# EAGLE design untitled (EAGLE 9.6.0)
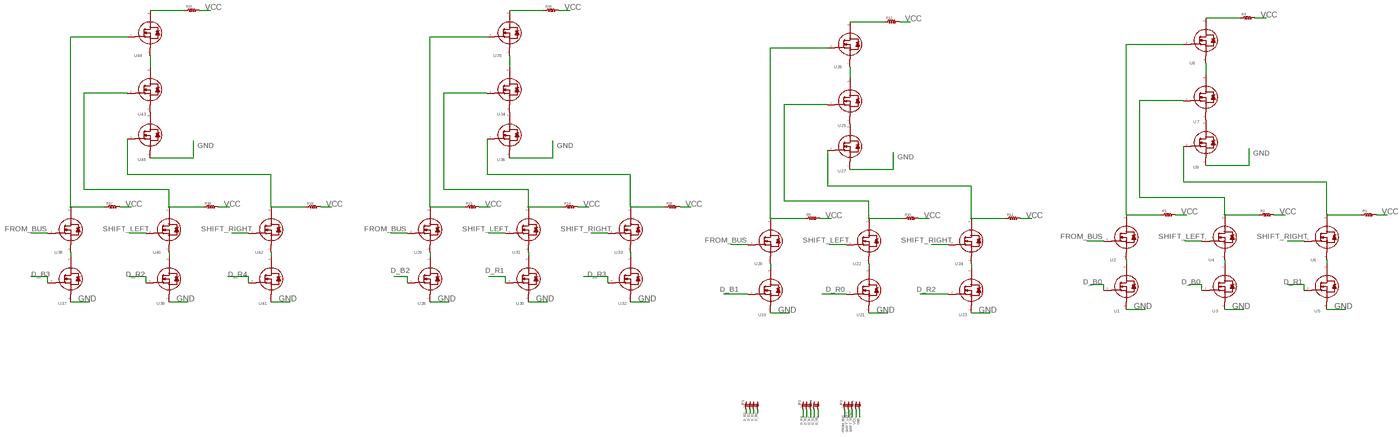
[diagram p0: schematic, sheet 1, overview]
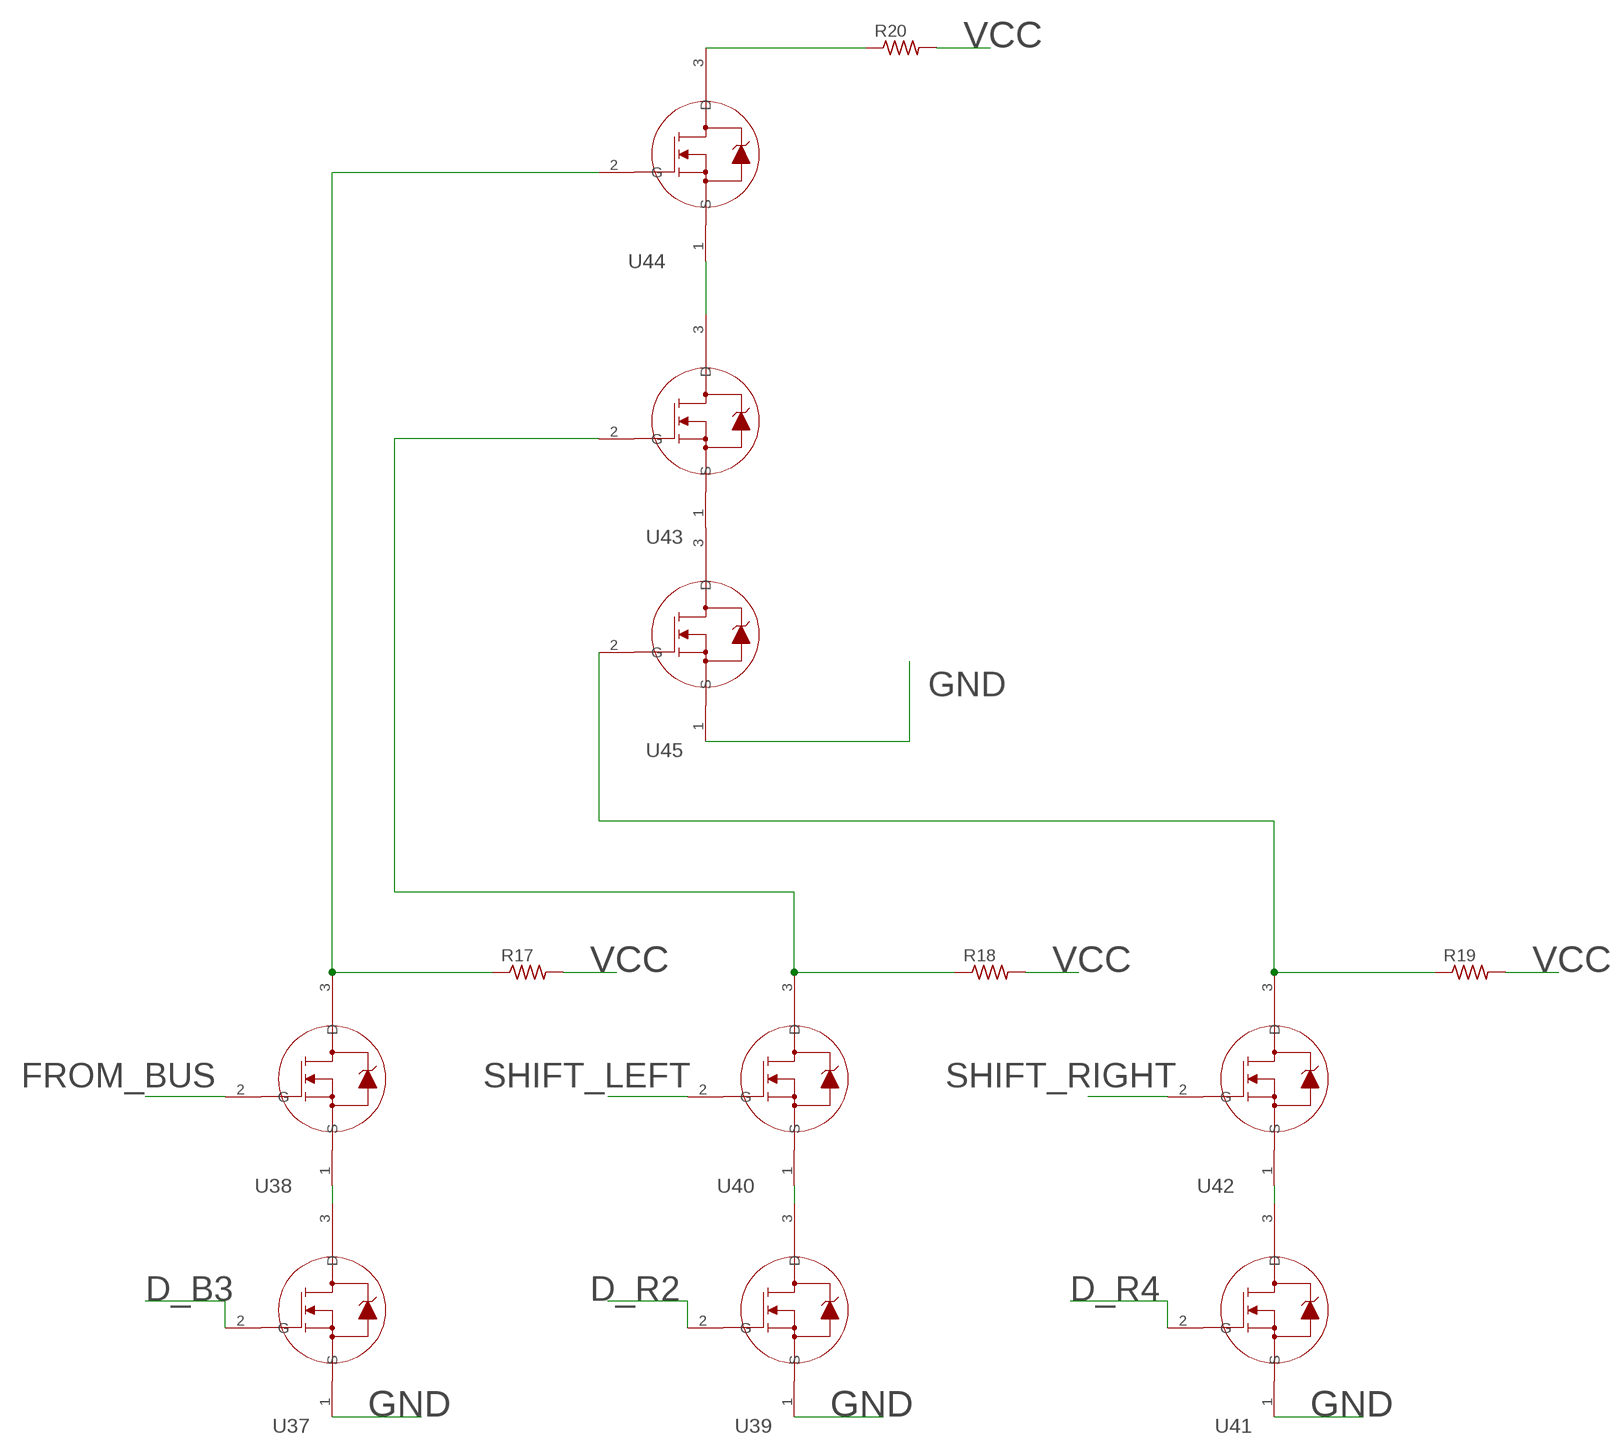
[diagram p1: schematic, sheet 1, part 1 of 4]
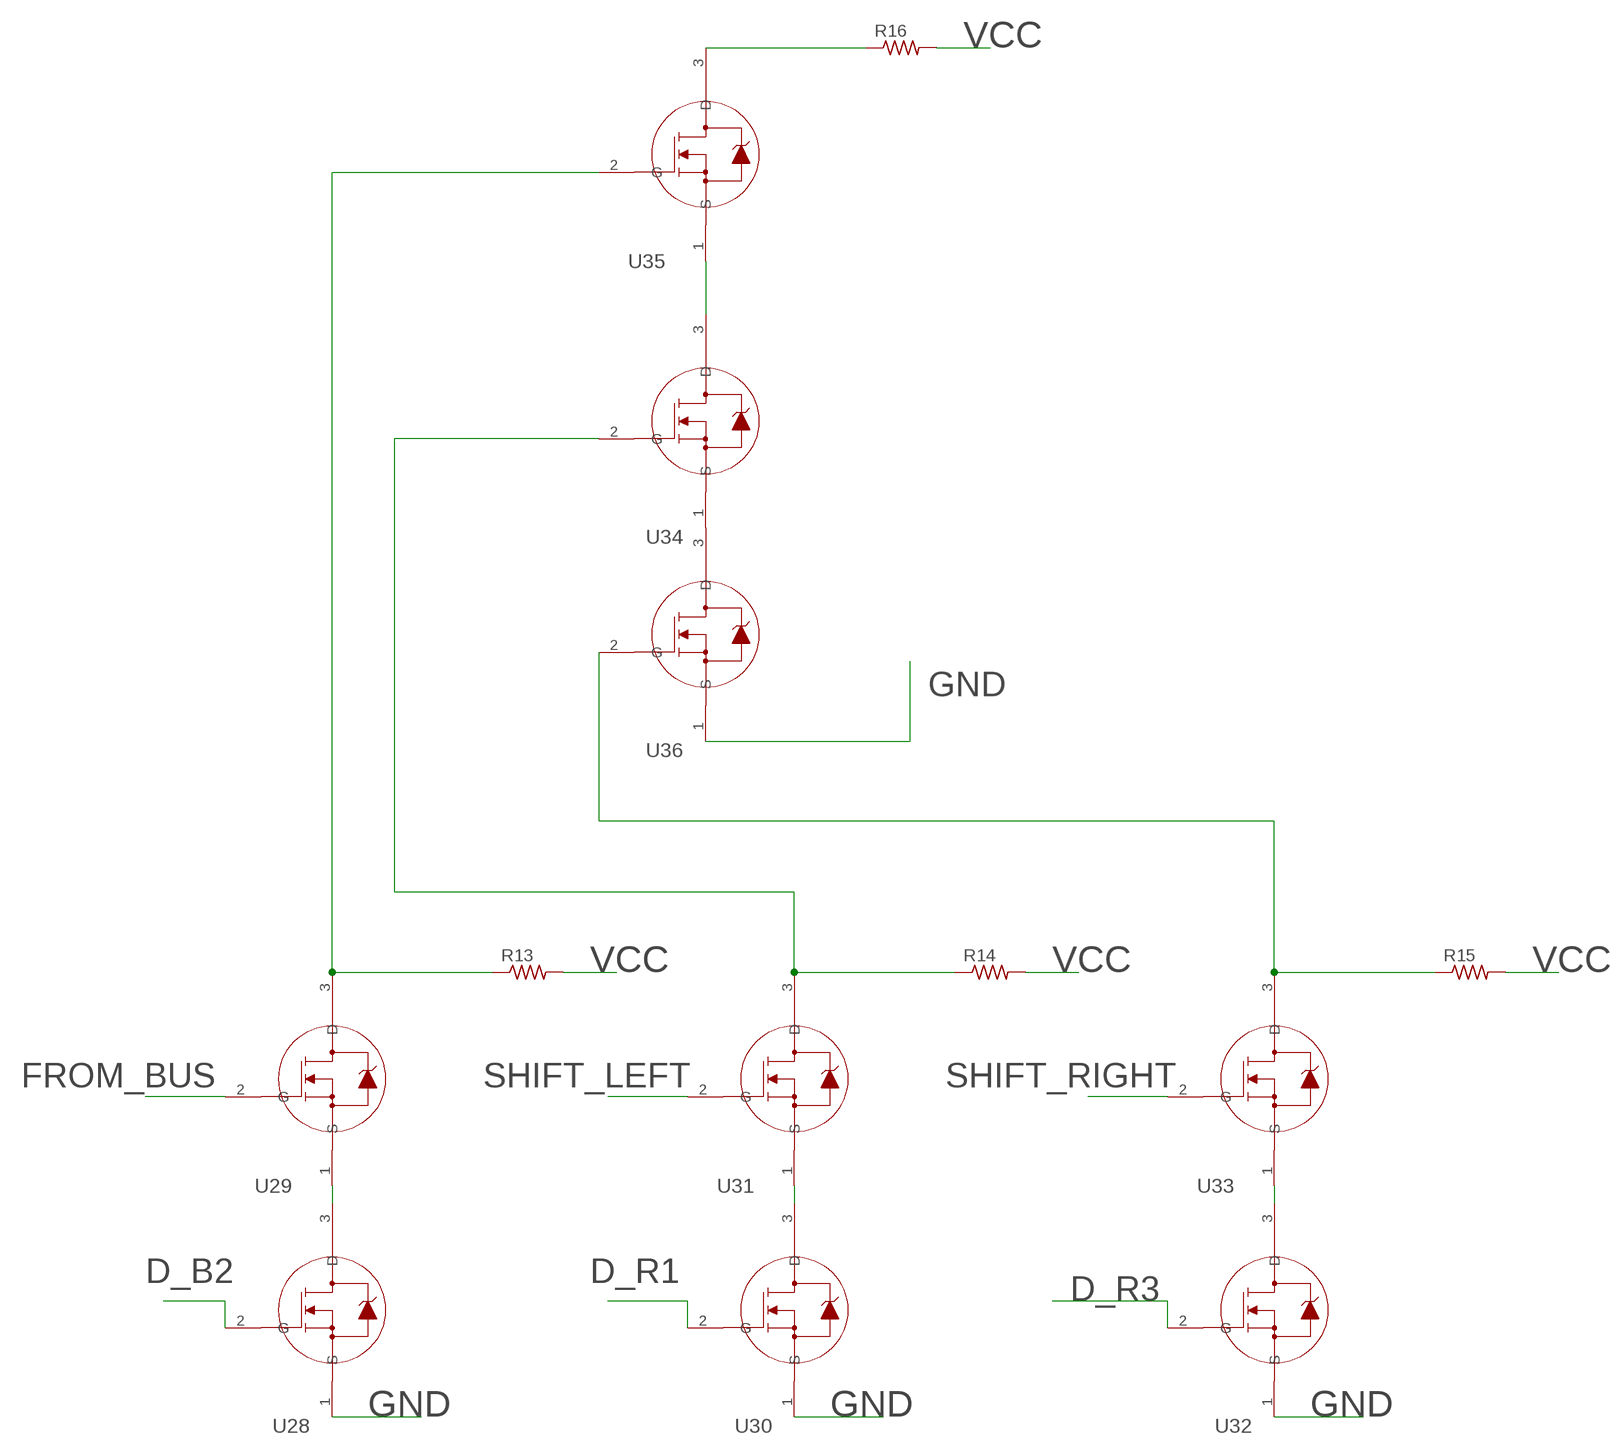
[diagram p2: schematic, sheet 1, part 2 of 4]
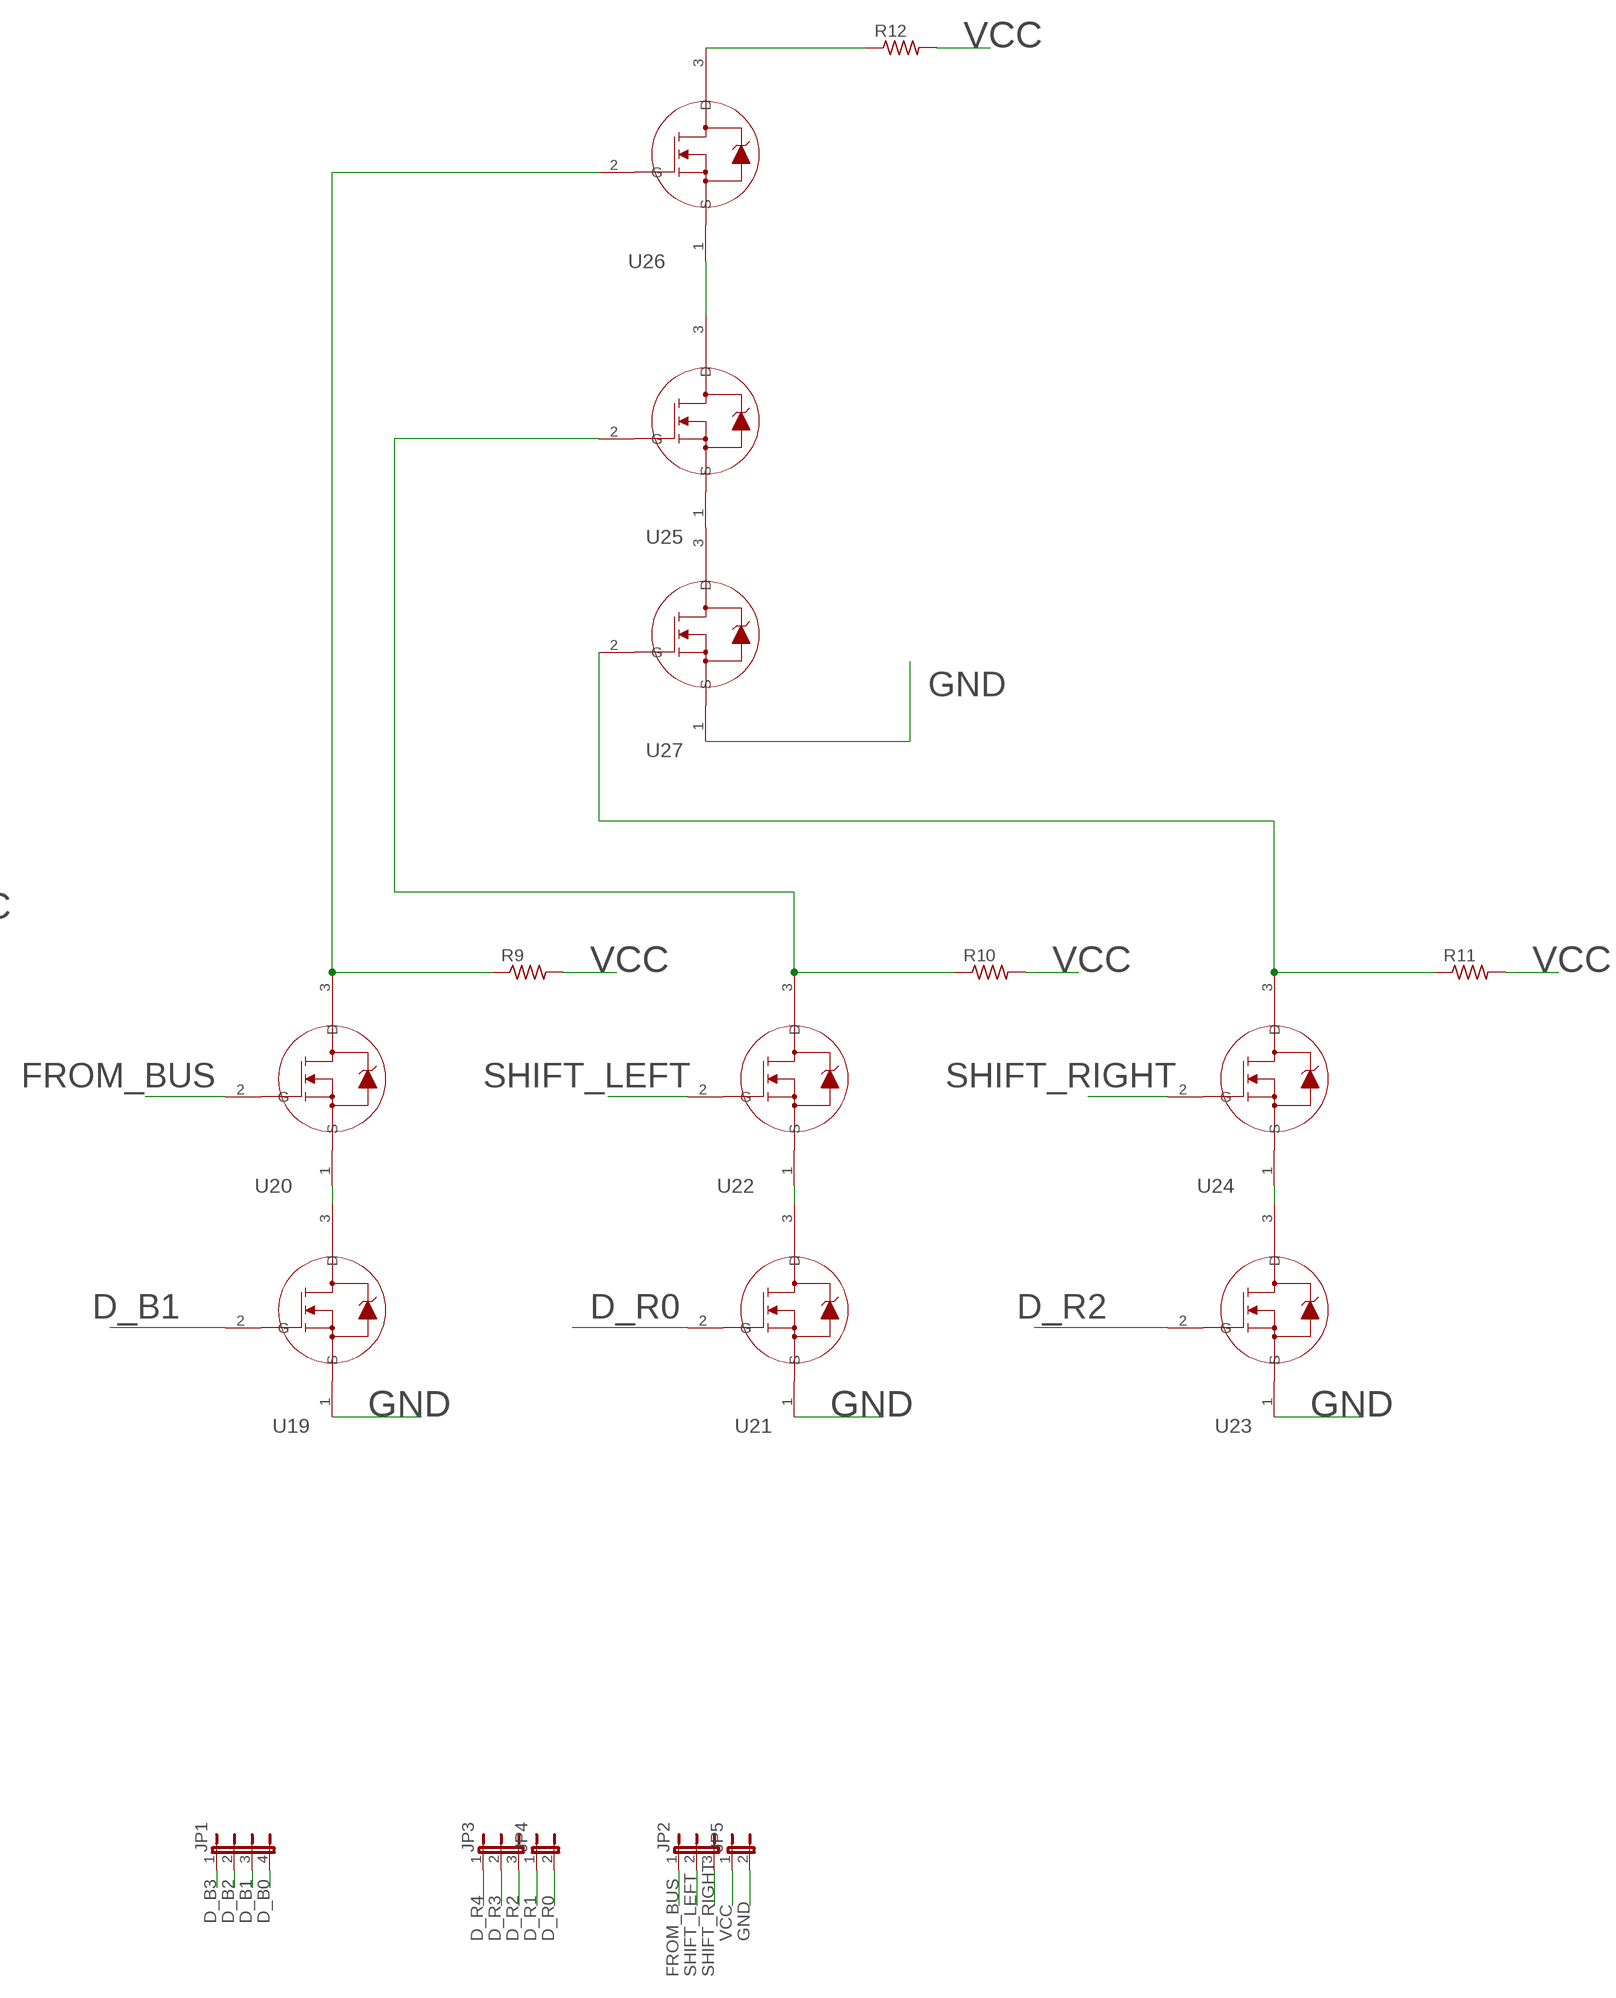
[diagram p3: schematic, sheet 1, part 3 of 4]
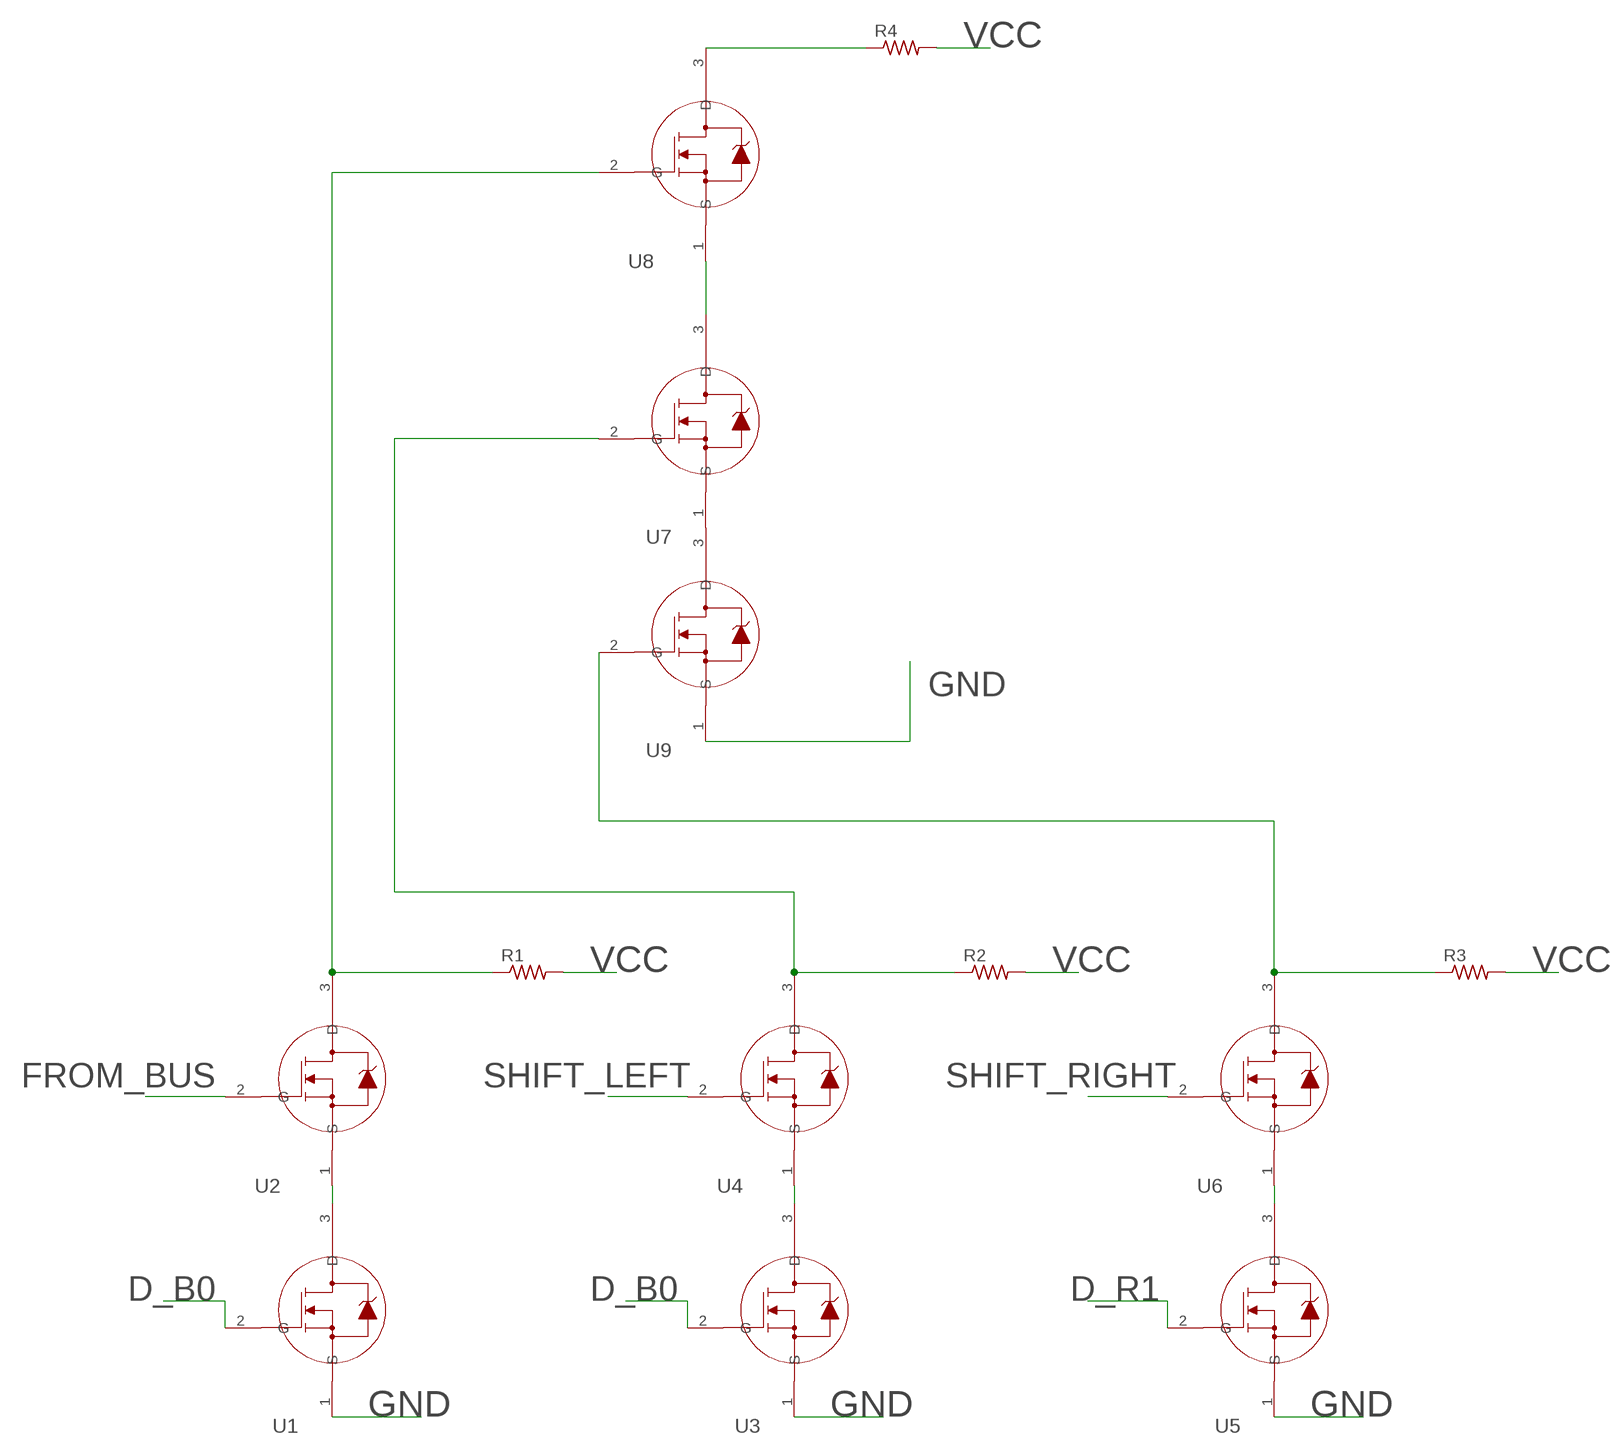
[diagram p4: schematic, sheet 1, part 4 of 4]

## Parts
JP1  JP4E  [JP4]
JP2  JP2E  [JP2]
JP3  JP2E  [JP2]
JP4  JP1E  [JP1]
JP5  JP1E  [JP1]
R1  R-US_0204/7  [0204/7]
R2  R-US_0204/7  [0204/7]
R3  R-US_0204/7  [0204/7]
R4  R-US_0204/7  [0204/7]
R9  R-US_0204/7  [0204/7]
R10  R-US_0204/7  [0204/7]
R11  R-US_0204/7  [0204/7]
R12  R-US_0204/7  [0204/7]
R13  R-US_0204/7  [0204/7]
R14  R-US_0204/7  [0204/7]
R15  R-US_0204/7  [0204/7]
R16  R-US_0204/7  [0204/7]
R17  R-US_0204/7  [0204/7]
R18  R-US_0204/7  [0204/7]
R19  R-US_0204/7  [0204/7]
R20  R-US_0204/7  [0204/7]
U1  2N7000RLRAG  [TO-92_ONS]
U2  2N7000RLRAG  [TO-92_ONS]
U3  2N7000RLRAG  [TO-92_ONS]
U4  2N7000RLRAG  [TO-92_ONS]
U5  2N7000RLRAG  [TO-92_ONS]
U6  2N7000RLRAG  [TO-92_ONS]
U7  2N7000RLRAG  [TO-92_ONS]
U8  2N7000RLRAG  [TO-92_ONS]
U9  2N7000RLRAG  [TO-92_ONS]
U19  2N7000RLRAG  [TO-92_ONS]
U20  2N7000RLRAG  [TO-92_ONS]
U21  2N7000RLRAG  [TO-92_ONS]
U22  2N7000RLRAG  [TO-92_ONS]
U23  2N7000RLRAG  [TO-92_ONS]
U24  2N7000RLRAG  [TO-92_ONS]
U25  2N7000RLRAG  [TO-92_ONS]
U26  2N7000RLRAG  [TO-92_ONS]
U27  2N7000RLRAG  [TO-92_ONS]
U28  2N7000RLRAG  [TO-92_ONS]
U29  2N7000RLRAG  [TO-92_ONS]
U30  2N7000RLRAG  [TO-92_ONS]
U31  2N7000RLRAG  [TO-92_ONS]
U32  2N7000RLRAG  [TO-92_ONS]
U33  2N7000RLRAG  [TO-92_ONS]
U34  2N7000RLRAG  [TO-92_ONS]
U35  2N7000RLRAG  [TO-92_ONS]
U36  2N7000RLRAG  [TO-92_ONS]
U37  2N7000RLRAG  [TO-92_ONS]
U38  2N7000RLRAG  [TO-92_ONS]
U39  2N7000RLRAG  [TO-92_ONS]
U40  2N7000RLRAG  [TO-92_ONS]
U41  2N7000RLRAG  [TO-92_ONS]
U42  2N7000RLRAG  [TO-92_ONS]
U43  2N7000RLRAG  [TO-92_ONS]
U44  2N7000RLRAG  [TO-92_ONS]
U45  2N7000RLRAG  [TO-92_ONS]

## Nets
D_B0: JP1.4 U1.2(G) U3.2(G)
D_B1: JP1.3 U19.2(G)
D_B2: JP1.2 U28.2(G)
D_B3: JP1.1 U37.2(G)
D_R0: JP4.2 U21.2(G)
D_R1: JP4.1 U5.2(G) U30.2(G)
D_R2: JP3.3 U23.2(G) U39.2(G)
D_R3: JP3.2 U32.2(G)
D_R4: JP3.1 U41.2(G)
FROM_BUS: JP2.1 U2.2(G) U20.2(G) U29.2(G) U38.2(G)
GND: JP5.2 U1.1(S) U3.1(S) U5.1(S) U9.1(S) U19.1(S) U21.1(S) U23.1(S) U27.1(S) U28.1(S) U30.1(S) U32.1(S) U36.1(S) U37.1(S) U39.1(S) U41.1(S) U45.1(S)
N$1: U1.3(D) U2.1(S)
N$2: R1.1 U2.3(D) U8.2(G)
N$3: U3.3(D) U4.1(S)
N$4: R2.1 U4.3(D) U7.2(G)
N$5: U5.3(D) U6.1(S)
N$6: R3.1 U6.3(D) U9.2(G)
N$7: U7.3(D) U8.1(S)
N$9: R4.1 U8.3(D)
N$11: U7.1(S) U9.3(D)
N$19: U19.3(D) U20.1(S)
N$20: R9.1 U20.3(D) U26.2(G)
N$21: U21.3(D) U22.1(S)
N$22: R10.1 U22.3(D) U25.2(G)
N$23: U23.3(D) U24.1(S)
N$24: R11.1 U24.3(D) U27.2(G)
N$25: U25.3(D) U26.1(S)
N$26: R12.1 U26.3(D)
N$27: U25.1(S) U27.3(D)
N$28: U28.3(D) U29.1(S)
N$29: R13.1 U29.3(D) U35.2(G)
N$30: U30.3(D) U31.1(S)
N$31: R14.1 U31.3(D) U34.2(G)
N$32: U32.3(D) U33.1(S)
N$33: R15.1 U33.3(D) U36.2(G)
N$34: U34.3(D) U35.1(S)
N$35: R16.1 U35.3(D)
N$36: U34.1(S) U36.3(D)
N$37: U37.3(D) U38.1(S)
N$38: R17.1 U38.3(D) U44.2(G)
N$39: U39.3(D) U40.1(S)
N$40: R18.1 U40.3(D) U43.2(G)
N$41: U41.3(D) U42.1(S)
N$42: R19.1 U42.3(D) U45.2(G)
N$43: U43.3(D) U44.1(S)
N$44: R20.1 U44.3(D)
N$45: U43.1(S) U45.3(D)
SHIFT_LEFT: JP2.2 U4.2(G) U22.2(G) U31.2(G) U40.2(G)
SHIFT_RIGHT: JP2.3 U6.2(G) U24.2(G) U33.2(G) U42.2(G)
VCC: JP5.1 R1.2 R2.2 R3.2 R4.2 R9.2 R10.2 R11.2 R12.2 R13.2 R14.2 R15.2 R16.2 R17.2 R18.2 R19.2 R20.2

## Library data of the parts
JP1 = jumper:JP4E: JUMPER
JP2 JP3 = jumper:JP2E: JUMPER
JP4 JP5 = jumper:JP1E: JUMPER
R1-R4 R9-R20 = rcl:R-US_: RESISTOR, American symbol; SPICEPREFIX: R
U1-U9 U19-U45 = Transistor(MOSFET):2N7000RLRAG; COPYRIGHT: Copyright (C) 2022 Ultra Librarian. All rights reserved.; MANUFACTURER_PART_NUMBER: 2N7000RLRAG; MFR_NAME: onsemi

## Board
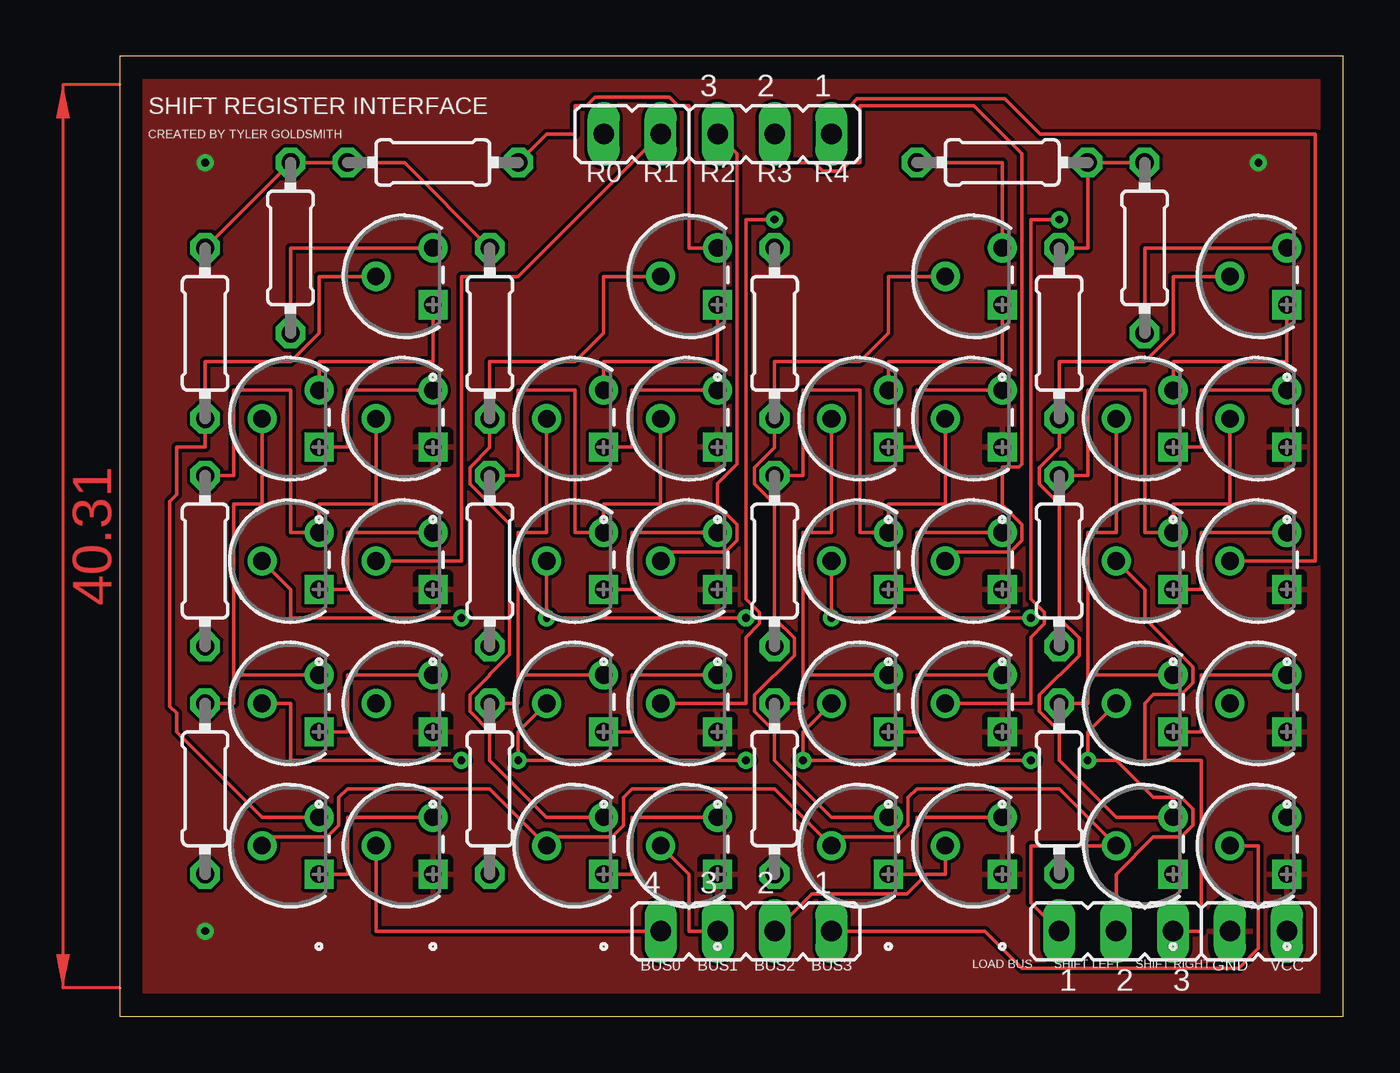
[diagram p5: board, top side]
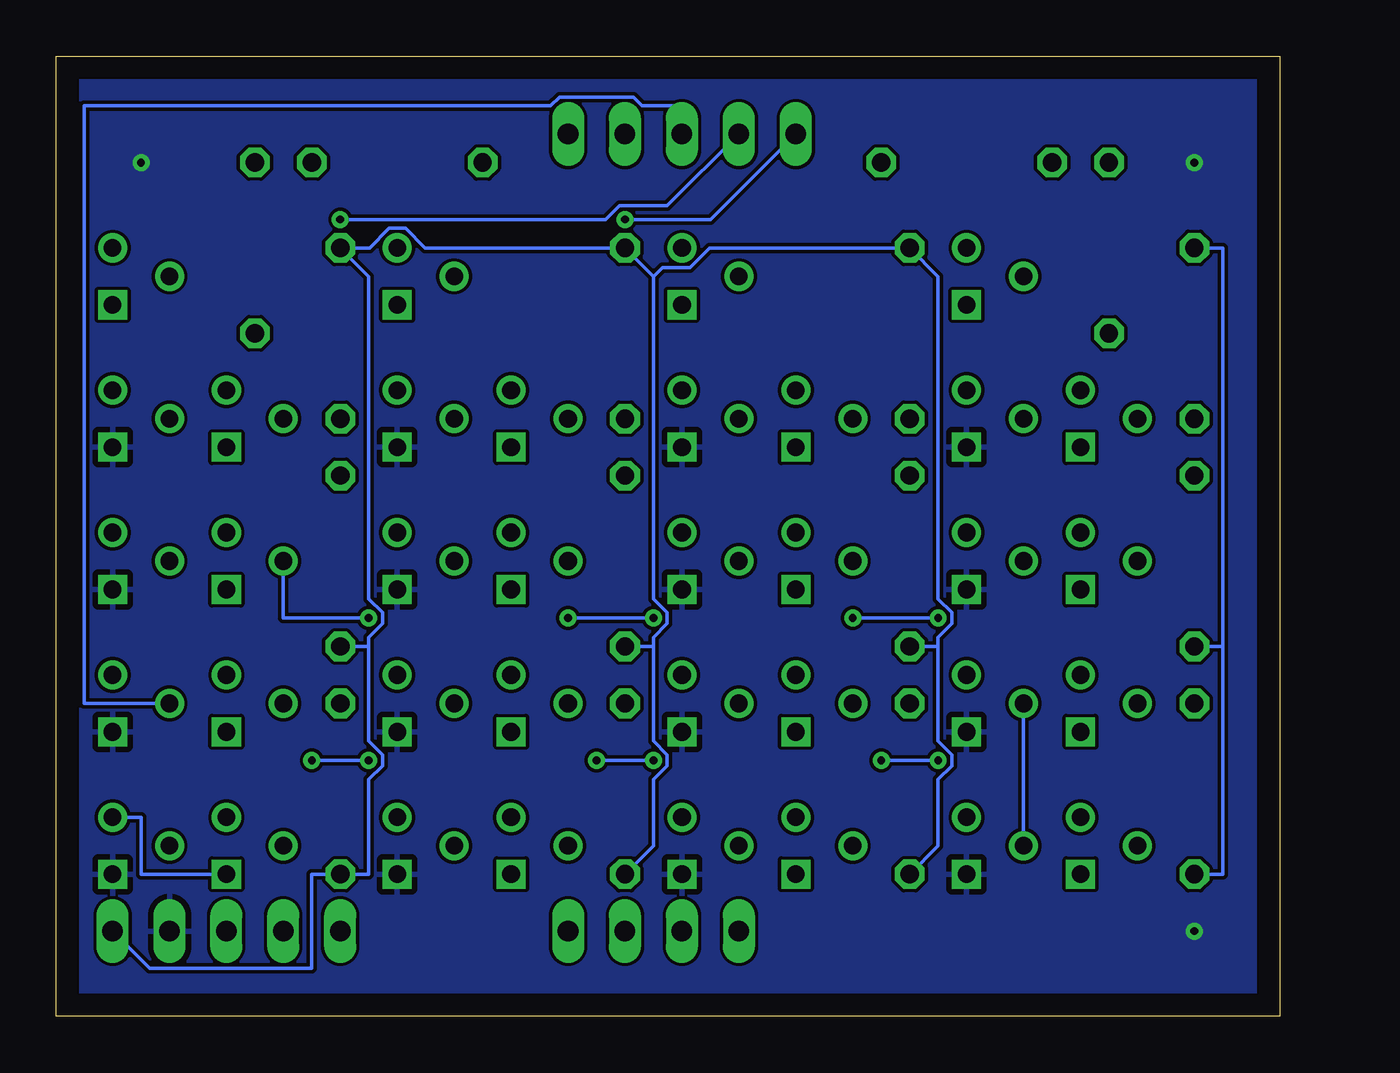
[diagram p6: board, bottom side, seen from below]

Size 54.59 x 42.85 mm. Coordinates in mm from the lower left corner, seen from the top.
Outline: 0,0 54.59,0 54.59,42.85 0,42.85 0,0
Copper layers (1*16): Top 0.035mm / dielectric 1.5mm / Bottom 0.035mm
Design rules "default": minimum track width 6mil, minimum drill 0.35mm, track to track 6mil, track to pad 6mil, pad to pad 6mil, via to via 6mil, smd to smd 6mil, copper to edge 40mil, drill to drill 6mil, minimum pad ring 10mil, minimum via ring 8mil, stop-mask expansion 4mil, vias tented up to drill 0mil, thermal gap 10mil

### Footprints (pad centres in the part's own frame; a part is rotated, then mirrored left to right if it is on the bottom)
JP4 = drill 0.914 long: 1 -3.81,0; 2 -1.27,0; 3 1.27,0; 4 3.81,0
JP2 = drill 0.914 long: 1 -2.54,0; 2 0,0; 3 2.54,0
JP1 = drill 0.914 long: 1 0,-1.27; 2 0,1.27
0204/7 = drill 0.813 octagon: 1 -3.81,0; 2 3.81,0
TO-92_ONS = drill 0.787 pad 1.295 square: 1 0,0 | drill 0.787 pad 1.295: 2 1.27,2.54; 3 2.54,0

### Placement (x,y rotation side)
JP1  27.94,3.81 180 top
JP2  44.45,3.81 0 top
JP3  29.21,39.37 180 top
JP4  22.86,39.37 90 top
JP5  50.8,3.81 90 top
R1  3.81,30.48 90 top
R2  3.81,10.16 270 top
R3  3.81,20.32 270 top
R4  7.62,34.29 90 top
R9  16.51,30.48 90 top
R10  16.51,10.16 270 top
R11  16.51,20.32 270 top
R12  13.97,38.1 180 top
R13  29.21,30.48 90 top
R14  29.21,10.16 270 top
R15  29.21,20.32 270 top
R16  39.37,38.1 0 top
R17  41.91,30.48 90 top
R18  41.91,10.16 270 top
R19  41.91,20.32 270 top
R20  45.72,34.29 90 top
U1  13.97,6.35 90 top
U2  8.89,6.35 90 top
U3  13.97,12.7 90 top
U4  8.89,12.7 90 top
U5  13.97,19.05 90 top
U6  8.89,19.05 90 top
U7  8.89,25.4 90 top
U8  13.97,31.75 90 top
U9  13.97,25.4 90 top
U19  26.67,6.35 90 top
U20  21.59,6.35 90 top
U21  26.67,12.7 90 top
U22  21.59,12.7 90 top
U23  26.67,19.05 90 top
U24  21.59,19.05 90 top
U25  21.59,25.4 90 top
U26  26.67,31.75 90 top
U27  26.67,25.4 90 top
U28  39.37,6.35 90 top
U29  34.29,6.35 90 top
U30  39.37,12.7 90 top
U31  34.29,12.7 90 top
U32  39.37,19.05 90 top
U33  34.29,19.05 90 top
U34  34.29,25.4 90 top
U35  39.37,31.75 90 top
U36  39.37,25.4 90 top
U37  52.07,6.35 90 top
U38  46.99,6.35 90 top
U39  52.07,12.7 90 top
U40  46.99,12.7 90 top
U41  52.07,19.05 90 top
U42  46.99,19.05 90 top
U43  46.99,25.4 90 top
U44  52.07,31.75 90 top
U45  52.07,25.4 90 top

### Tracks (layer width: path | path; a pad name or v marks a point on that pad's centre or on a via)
D_B0
  Top 0.152: U1.2 11.43,3.81 JP1.4
  Bottom 0.152: U1.2 U3.2
D_B1
  Top 0.152: U19.2 25.4,6.35 25.4,3.81 JP1.3
D_B2
  Top 0.152: U28.2 36.83,6.35 35.99,6.35 35.11,5.47 30.87,5.47 JP1.2
D_B3
  Top 0.152: JP1.1 38.6,3.81 40.25,2.16 49.92,2.16 50.8,3.04 50.8,7.62 U37.2
D_R0  (via drill 0.35)
  Top 0.152: U21.2 27.94,13.97 27.94,16.92 28.55,17.53 28.55,18.03 27.94,18.64 27.94,35.56 v29.21,35.56
  Bottom 0.152: v29.21,35.56 25.4,35.56 JP4.2
D_R1  (via drill 0.35)
  Top 0.152: U5.2 15.24,20.32 15.24,33.02 17.78,33.02 JP4.1 | U30.2 40.64,13.97 40.64,16.92 41.25,17.53 41.25,18.03 40.64,18.64 40.64,35.56 v41.91,35.56
  Bottom 0.152: JP4.1 27.33,36.17 29.46,36.17 30.07,35.56 v41.91,35.56
D_R2
  Top 0.152: U23.2 24.52,20.71 27.03,20.71 27.55,21.23 27.55,21.95 26.67,22.83 26.67,23.78 27.55,24.66 27.55,38.49 JP3.3
  Bottom 0.152: U39.2 53.34,13.97 53.34,40.64 32.52,40.64 32.14,41.02 28.82,41.02 28.44,40.64 26.67,40.64 JP3.3
D_R3
  Top 0.152: JP3.2 29.21,38.1 30.98,38.1 31.36,37.72 32.14,37.72 32.52,38.1 33.02,38.1 33.02,40.64 38.1,40.64 40.25,38.49 40.25,24.66 40.11,24.52 39.37,24.52 39.37,22.83 40.25,21.95 40.25,21.23 39.73,20.71 37.22,20.71 U32.2
D_R4
  Top 0.152: U41.2 53.34,20.32 53.34,39.37 41.07,39.37 39.5,40.95 32.89,40.95 32.59,40.64 31.75,40.64 JP3.1
FROM_BUS
  Top 0.152: U2.2 6.74,8.01 9.25,8.01 9.77,8.53 9.77,9.77 10.16,10.16 16.51,10.16 U20.2 19.44,8.01 21.95,8.01 22.47,8.53 22.47,9.77 22.86,10.16 29.21,10.16 U29.2 32.14,8.01 34.65,8.01 35.17,8.53 35.17,9.77 35.56,10.16 41.91,10.16 U38.2 40.64,7.62 40.64,5.08 JP2.1
GND  (via drill 0.35)
  other vias: 3.81,3.81 3.81,38.1 50.8,38.1
  pour Bottom: -6.35,44.45 57.15,44.45 57.15,-1.27 -6.35,-1.27
  pour Top: -6.35,44.45 57.15,44.45 57.15,-1.27 -6.35,-1.27
N$1
  Top 0.152: U2.1 10.16,6.35 10.16,8.89 U1.3
N$2
  Top 0.152: U8.2 8.89,33.02 8.89,30.48 7.62,29.21 3.81,29.21 R1.1 3.81,25.4 2.54,25.4 2.54,23.29 2.23,22.99 2.23,13.84 2.54,13.54 2.54,12.7 6.35,8.89 U2.3
N$3
  Top 0.152: U4.1 10.16,12.7 10.16,15.24 U3.3
N$4
  Top 0.152: R2.1 5.08,13.97 5.08,15.24 | 5.08,15.24 U4.3 | U7.2 6.35,22.86 5.08,22.86 5.08,15.24
N$5
  Top 0.152: U6.1 10.16,19.05 10.16,21.59 U5.3
N$6
  Top 0.152: U9.2 11.43,22.86 8.89,22.86 U6.3 7.62,21.59 7.62,27.94 5.08,27.94 5.08,24.13 R3.1
N$7
  Top 0.152: U7.3 8.89,29.21 13.97,29.21 U8.1
N$9
  Top 0.152: R4.1 7.62,34.29 U8.3
N$11
  Top 0.152: U7.1 10.16,25.4 10.16,27.94 U9.3
N$19
  Top 0.152: U20.1 22.86,6.35 22.86,8.89 U19.3
N$20
  Top 0.152: U26.2 21.59,33.02 21.59,30.48 20.32,29.21 16.51,29.21 R9.1 16.51,25.39 15.62,24.5 15.62,23.75 17.4,21.97 17.4,16.14 16.51,15.25 16.51,15.23 15.62,14.34 15.62,13.6 16.51,12.71 16.51,11.43 19.05,8.89 U20.3
N$21
  Top 0.152: U22.1 22.86,12.7 22.86,15.24 U21.3
N$22
  Top 0.152: R10.1 17.78,13.97 17.78,15.24 | U22.3 17.78,15.24 | 17.78,15.24 17.78,21.59 19.05,21.59 U25.2
N$23
  Top 0.152: U24.1 22.86,19.05 22.86,21.59 U23.3
N$24
  Top 0.152: U27.2 24.13,22.86 21.59,22.86 U24.3 20.32,21.59 20.32,27.94 17.78,27.94 17.78,24.13 R11.1
N$25
  Top 0.152: U25.3 21.59,29.21 26.67,29.21 U26.1
N$26
  Top 0.152: R12.1 19.05,39.37 20.32,39.37 20.32,40.64 20.82,40.64 21.2,41.02 24.52,41.02 24.9,40.64 25.4,40.64 25.4,34.29 U26.3
N$27
  Top 0.152: U25.1 22.86,25.4 22.86,27.94 U27.3
N$28
  Top 0.152: U29.1 35.56,6.35 35.56,8.89 U28.3
N$29
  Top 0.152: U35.2 34.29,33.02 34.29,30.48 33.02,29.21 29.21,29.21 R13.1 29.21,25.39 28.32,24.5 28.32,23.76 29.21,22.87 29.21,17.77 30.1,16.88 30.1,16.12 28.32,14.34 28.32,13.6 29.21,12.71 29.21,11.43 31.75,8.89 U29.3
N$30
  Top 0.152: U31.1 35.56,12.7 35.56,15.24 U30.3
N$31
  Top 0.152: R14.1 30.48,13.97 30.48,15.24 | 30.48,15.24 U31.3 | 30.48,15.24 30.48,21.59 31.75,21.59 U34.2
N$32
  Top 0.152: U33.1 35.56,19.05 35.56,21.59 U32.3
N$33
  Top 0.152: U36.2 36.83,22.86 34.29,22.86 U33.3 33.02,21.59 33.02,27.94 30.48,27.94 30.48,24.13 R15.1
N$34
  Top 0.152: U34.3 34.29,29.21 39.37,29.21 U35.1
N$35
  Top 0.152: R16.1 39.37,38.1 U35.3
N$36
  Top 0.152: U34.1 35.56,25.4 35.56,27.94 U36.3
N$37
  Bottom 0.152: U38.1 50.8,6.35 50.8,8.89 U37.3
N$38
  Top 0.152: U44.2 46.99,33.02 46.99,30.48 45.72,29.21 41.91,29.21 R17.1 41.91,25.39 41.02,24.5 41.02,23.76 41.91,22.87 41.91,17.77 42.8,16.88 42.8,16.12 41.02,14.34 41.02,13.6 41.91,12.71 41.91,11.43 44.45,8.89 U38.3
N$39
  Top 0.152: U40.1 48.26,12.7 48.26,15.24 U39.3
N$40
  Top 0.152: R18.1 43.18,13.97 43.18,15.24 | 43.18,15.24 U40.3 | 43.18,15.24 43.18,21.59 44.45,21.59 U43.2
N$41
  Top 0.152: U42.1 48.26,19.05 48.26,21.59 U41.3
N$42
  Top 0.152: U45.2 49.53,22.86 46.99,22.86 U42.3 45.72,21.59 45.72,27.94 43.18,27.94 43.18,24.13 R19.1
N$43
  Top 0.152: U43.3 46.99,29.21 52.07,29.21 U44.1
N$44
  Top 0.152: R20.1 45.72,34.29 U44.3
N$45
  Top 0.152: U43.1 48.26,25.4 48.26,27.94 U45.3
SHIFT_LEFT  (via drill 0.35)
  Top 0.152: U4.2 7.62,13.97 7.62,11.43 v15.24,11.43 | U22.2 17.78,12.7 v17.78,11.43 v27.94,11.43 | U31.2 30.48,12.7 v30.48,11.43 v40.64,11.43 | U40.2 43.18,12.7 v43.18,11.43 44.45,11.43 46.11,9.77 47.35,9.77 47.87,9.25 47.87,8.53 47.35,8.01 46.11,8.01 44.45,6.35 JP2.2
  Bottom 0.152: v15.24,11.43 v17.78,11.43 | v27.94,11.43 v30.48,11.43 | v40.64,11.43 v43.18,11.43
SHIFT_RIGHT  (via drill 0.35)
  Top 0.152: U6.2 7.62,19.05 7.62,17.78 v15.24,17.78 | U24.2 v19.05,17.78 v27.94,17.78 | U33.2 v31.75,17.78 v40.64,17.78 | JP2.3 48.26,3.81 48.26,11.43 45.72,11.43 45.72,13.97 46.11,14.36 47.35,14.36 47.87,14.88 47.87,15.6 45.72,17.75 45.72,19.05 U42.2
  Bottom 0.152: v15.24,17.78 v19.05,17.78 | v27.94,17.78 v31.75,17.78 | v40.64,17.78 44.45,17.78 U42.2
VCC
  Top 0.152: R9.2 12.7,38.1 R12.2 R4.2 R1.2 | R17.2 43.18,34.29 R16.2 R20.2
  Bottom 0.152: R1.2 2.54,34.29 2.54,16.51 | 2.54,16.51 R3.2 | R2.2 2.54,6.35 2.54,16.51 | R11.2 15.24,16.51 | 15.24,16.51 15.24,16.92 14.63,17.53 14.63,18.03 15.24,18.64 15.24,33.02 R9.2 25.43,34.29 26.31,33.41 27.55,33.41 27.94,33.02 | 15.24,16.51 15.24,12.29 14.63,11.68 14.63,11.18 15.24,10.57 15.24,7.62 R10.2 | R14.2 27.94,7.62 27.94,10.57 27.33,11.18 27.33,11.68 27.94,12.29 27.94,16.51 | 27.94,16.51 R15.2 | 27.94,16.51 27.94,16.92 27.33,17.53 27.33,18.03 27.94,18.64 27.94,33.02 | 27.94,33.02 R13.2 38.13,34.29 39.01,35.17 39.73,35.17 40.61,34.29 R17.2 40.64,33.02 40.64,18.64 40.03,18.03 40.03,17.53 40.64,16.92 40.64,16.51 | R19.2 40.64,16.51 | 40.64,16.51 40.64,12.29 40.03,11.68 40.03,11.18 40.64,10.57 40.64,6.35 R18.2 43.18,6.35 43.18,2.16 50.42,2.16 JP5.1
(copper drawn outside any net)
  shapes: Top area x1

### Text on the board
tNames: SHIFT REGISTER INTERFACE | CREATED BY TYLER GOLDSMITH | R0 | R1 | R2 | R3 | R4 | BUS0 | BUS1 | BUS2 | BUS3 | LOAD BUS | SHIFT LEFT | SHIFT RIGHT | GND | VCC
